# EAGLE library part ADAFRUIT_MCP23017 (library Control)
http://ww1.microchip.com/downloads/en/DeviceDoc/21952a.pdf Source: http://ww1.microchip.com/downloads/en/DeviceDoc/21952a.pdf
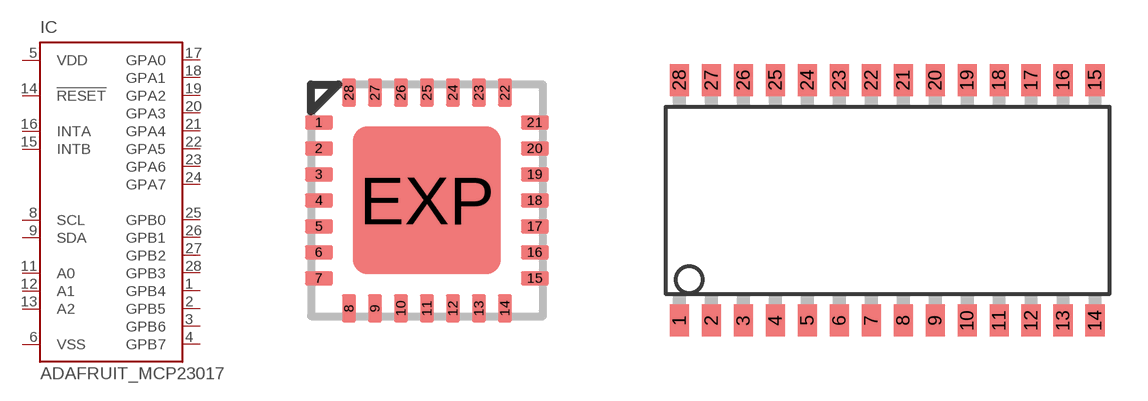
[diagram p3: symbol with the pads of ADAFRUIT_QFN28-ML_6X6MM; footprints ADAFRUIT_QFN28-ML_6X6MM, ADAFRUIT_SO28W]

Designator prefix IC

## ADAFRUIT_MCP23017ML  [ADAFRUIT_QFN28-ML_6X6MM]
1  GPB4
2  GPB5
3  GPB6
4  GPB7
5  VDD  pwr
6  VSS  pwr
8  SCL  in
9  SDA
11  A0  in
12  A1  in
13  A2  in
14  !RESET  in
15  INTB  out
16  INTA  out
17  GPA0
18  GPA1
19  GPA2
20  GPA3
21  GPA4
22  GPA5
23  GPA6
24  GPA7
25  GPB0
26  GPB1
27  GPB2
28  GPB3

## ADAFRUIT_MCP23017SO  [ADAFRUIT_SO28W]
1  GPB0
2  GPB1
3  GPB2
4  GPB3
5  GPB4
6  GPB5
7  GPB6
8  GPB7
9  VDD  pwr
10  VSS  pwr
12  SCL  in
13  SDA
15  A0  in
16  A1  in
17  A2  in
18  !RESET  in
19  INTB  out
20  INTA  out
21  GPA0
22  GPA1
23  GPA2
24  GPA3
25  GPA4
26  GPA5
27  GPA6
28  GPA7

## ADAFRUIT_MCP23017SP  [ADAFRUIT_DIL28-3]
Pads as for ADAFRUIT_SO28W

## ADAFRUIT_MCP23017SP2  [ADAFRUIT_DIL28-3-ROUND]
Pads as for ADAFRUIT_SO28W

## ADAFRUIT_MCP23017SS  [ADAFRUIT_SSOP28]
Pads as for ADAFRUIT_SO28W

## Footprint ADAFRUIT_QFN28-ML_6X6MM (pad centres in mm)
QFN28-ML_6X6MM Source: http://www.microchip.com .. 39637a.pdf
smd 0.7 x 0.35: 1 -2.7,1.95; 2 -2.7,1.3; 3 -2.7,0.65; 4 -2.7,0; 5 -2.7,-0.65; 6 -2.7,-1.3; 7 -2.7,-1.95; 15 2.7,-1.95; 16 2.7,-1.3; 17 2.7,-0.65; 18 2.7,0; 19 2.7,0.65; 20 2.7,1.3; 21 2.7,1.95
smd 0.35 x 0.7: 8 -1.95,-2.7; 9 -1.3,-2.7; 10 -0.65,-2.7; 11 0,-2.7; 12 0.65,-2.7; 13 1.3,-2.7; 14 1.95,-2.7; 22 1.95,2.7; 23 1.3,2.7; 24 0.65,2.7; 25 0,2.7; 26 -0.65,2.7; 27 -1.3,2.7; 28 -1.95,2.7
smd 3.7 x 3.7: EXP 0,0

## Footprint ADAFRUIT_SO28W (pad centres in mm)
28-Lead Plastic Small Outline (SO) Wide, 300 mil Body (SOIC) Source: http://ww1.microchip.com/downloads/en/devicedoc/39632c.pdf
smd 0.762 x 1.27: 1 -7.62,-4.78; 2 -6.35,-4.78; 3 -5.08,-4.78; 4 -3.81,-4.78; 5 -2.54,-4.78; 6 -1.27,-4.78; 7 0,-4.78; 8 1.27,-4.78; 9 2.54,-4.78; 10 3.81,-4.78; 11 5.08,-4.78; 12 6.35,-4.78; 13 7.62,-4.78; 14 8.89,-4.78; 15 8.89,4.78; 16 7.62,4.78; 17 6.35,4.78; 18 5.08,4.78; 19 3.81,4.78; 20 2.54,4.78; 21 1.27,4.78; 22 0,4.78; 23 -1.27,4.78; 24 -2.54,4.78; 25 -3.81,4.78; 26 -5.08,4.78; 27 -6.35,4.78; 28 -7.62,4.78

## Footprint ADAFRUIT_DIL28-3 (pad centres in mm)
Dual In Line package type P
drill 0.813 long: 1 -16.51,-3.81; 2 -13.97,-3.81; 3 -11.43,-3.81; 4 -8.89,-3.81; 5 -6.35,-3.81; 6 -3.81,-3.81; 7 -1.27,-3.81; 8 1.27,-3.81; 9 3.81,-3.81; 10 6.35,-3.81; 11 8.89,-3.81; 12 11.43,-3.81; 13 13.97,-3.81; 14 16.51,-3.81; 15 16.51,3.81; 16 13.97,3.81; 17 11.43,3.81; 18 8.89,3.81; 19 6.35,3.81; 20 3.81,3.81; 21 1.27,3.81; 22 -1.27,3.81; 23 -3.81,3.81; 24 -6.35,3.81; 25 -8.89,3.81; 26 -11.43,3.81; 27 -13.97,3.81; 28 -16.51,3.81

## Footprint ADAFRUIT_DIL28-3-ROUND (pad centres in mm)
drill 0.813 pad 1.676: 1 -16.51,-3.81; 2 -13.97,-3.81; 3 -11.43,-3.81; 4 -8.89,-3.81; 5 -6.35,-3.81; 6 -3.81,-3.81; 7 -1.27,-3.81; 8 1.27,-3.81; 9 3.81,-3.81; 10 6.35,-3.81; 11 8.89,-3.81; 12 11.43,-3.81; 13 13.97,-3.81; 14 16.51,-3.81; 15 16.51,3.81; 16 13.97,3.81; 17 11.43,3.81; 18 8.89,3.81; 19 6.35,3.81; 20 3.81,3.81; 21 1.27,3.81; 22 -1.27,3.81; 23 -3.81,3.81; 24 -6.35,3.81; 25 -8.89,3.81; 26 -11.43,3.81; 27 -13.97,3.81; 28 -16.51,3.81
